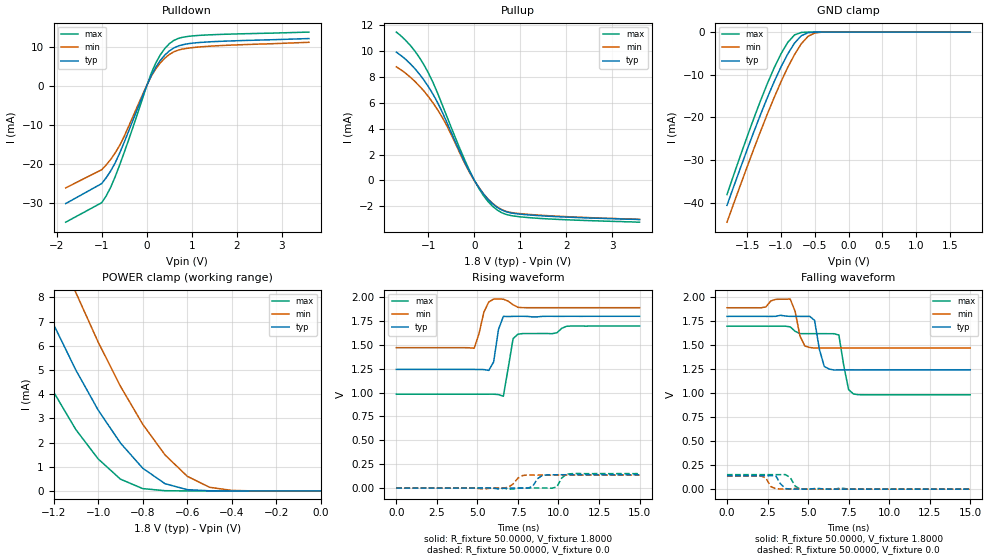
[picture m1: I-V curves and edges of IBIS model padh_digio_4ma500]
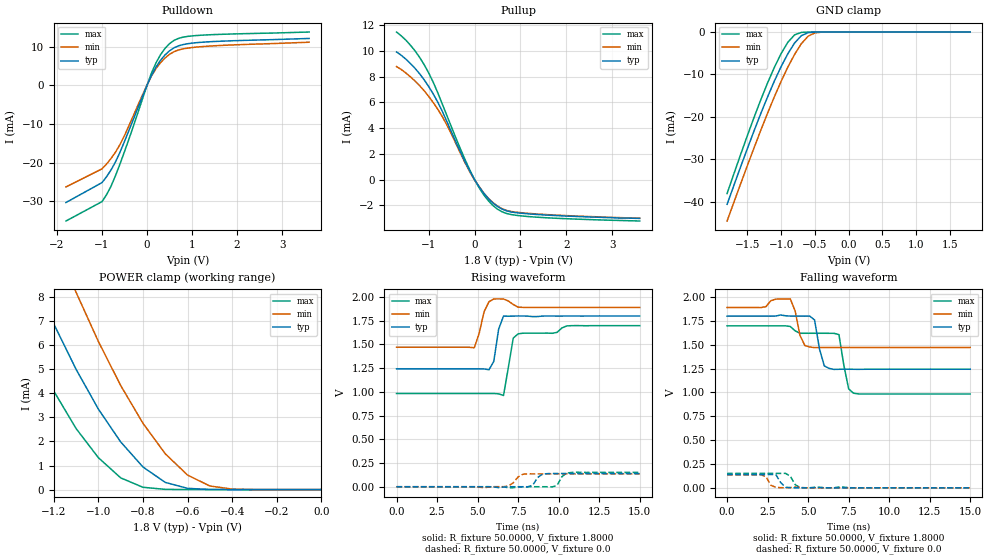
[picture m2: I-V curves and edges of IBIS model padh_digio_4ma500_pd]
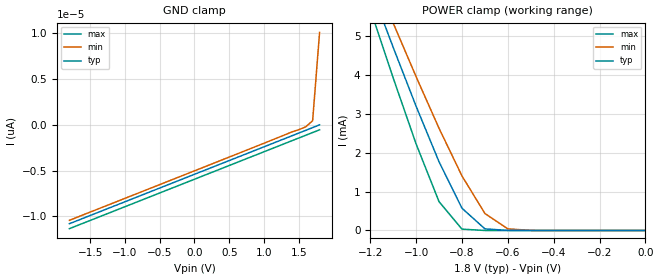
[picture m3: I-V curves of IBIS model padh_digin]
| IBIS file cs4272.ibs created by s2ibis3 verion 1.0
| North Carolina State University, ERL, 2005
[IBIS ver]   3.2
[Comment char]  |_char
[File name]   cs4272.ibs
[File Rev]   1.0B
[Date]   January 26, 2003
[Source]   HSpice Netlist
[Notes]   Rev. 1.0  1/26/2006  28-pin.  Original file.
|   Created by D. DeVries
[Copyright]   (C)opyright 2003 Cirrus Logic, Inc.  All Rights Reserved
[Component]   cs4272
[Manufacturer]  Cirrus Logic, Inc.
|   Component cs4272
[Package]
| variable   typ   min   max
R_pkg   12m   6.8m   16.1m
L_pkg   1.4n   0.713n   2.100n
C_pkg   0.27p   0.180p   0.368p
[Pin]  signal_name   model_name   R_pin   L_pin   C_pin
1   XTO   NC
2   XTI   NC
3   MCLK   padh_digio_mclk_pd
4   LRCK   padh_digio_4ma500
5   SCLK   padh_digio_4ma500
6   SDOUT   padh_digio_4ma500_pd
7   SDIN   padh_digin
8   DGND   GND
9   VD   POWER
10   VL   POWER
11   SCL_CCLK   padh_digin
12   SDA_CDIN   padh_digio_mclk
13   AD0_CSB   padh_digin
14   RSTB   padh_digin
15   VCOM   NC
16   AINA-   NC
17   AINA+   NC
18   AINB+   NC
19   AINB-   NC
20   VA   POWER
21   AGND   GND
22   FILT+   NC
23   AMUTECB   NC
24   AOUTA-   NC
25   AOUTA+   NC
26   AOUTB+   NC
27   AOUTB-   NC
28   BMUTECB   NC
| Models and submodels in the file (5): padh_digio_4ma500 (I/O), padh_digio_4ma500_pd (I/O), padh_digin (Input), padh_digio_mclk (I/O), padh_digio_mclk_pd (I/O)
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|   Model sclk
[Model]  padh_digio_4ma500
Model_type I/O
Polarity   Non-Inverting
Enable   Active-High
Vinl =   0.625V
Vinh =   0.975V
C_comp   5.0000pF   5.0000pF   5.0000pF
[Temperature Range]   25.0000   85.0000   -40.0000
[Voltage Range]   1.8000V   1.6200V   1.9800V
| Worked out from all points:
|   slope of the pulldown table from 0 to 0.27 V, typ, clamps not added: 45.5 ohm
|   slope of the pullup table from 0 to 0.27 V, typ, clamps not added: 199 ohm
|   GND clamp passes 1 mA (typ) near -0.71 V on its own axis
|   POWER clamp passes 1 mA (typ) near -0.81 V on its own axis
|   rising waveform, R_fixture 50.0000, V_fixture 1.8000: 20-80 % time 329ps typ, 374ps min, 423ps max; typ from 1.24 V to 1.8 V
|   rising waveform, R_fixture 50.0000, V_fixture 0.0: 20-80 % time 378ps typ, 473ps min, 360ps max; typ from 0 V to 0.139 V
|   falling waveform, R_fixture 50.0000, V_fixture 1.8000: 20-80 % time 401ps typ, 363ps min, 445ps max; typ from 1.8 V to 1.24 V
|   falling waveform, R_fixture 50.0000, V_fixture 0.0: 20-80 % time 366ps typ, 272ps min, 323ps max; typ from 0.139 V to 0 V
[Pulldown]
|Voltage   I(typ)   I(min)   I(max)
-1.8V     -30.27mA   -26.24mA   -35.05mA
-1V       -25.14mA   -21.58mA   -30.05mA
-900mV    -23.63mA   -20.35mA   -28.29mA
-800mV    -21.88mA   -18.91mA   -26.07mA
-600mV    -17.28mA   -15.3mA    -20.3mA
0V        -4.47pA    55.01uA    80fA
100mV     2.574mA    2.437mA    3.196mA
300mV     6.46mA     5.835mA    7.9mA
500mV     8.908mA    7.999mA    10.75mA
700mV     10.19mA    9.127mA    12.12mA
1.1V      11.01mA    9.864mA    12.85mA
3.6V      12.09mA    11.13mA    13.75mA
[Pullup]
|Voltage   I(typ)   I(min)   I(max)
-1.7V     9.93mA     8.79mA     11.48mA
-1.4V     9.04mA     8mA        10.47mA
-1.1V     7.773mA    6.922mA    8.954mA
-900mV    6.661mA    5.992mA    7.572mA
-700mV    5.289mA    4.882mA    5.856mA
-300mV    2.086mA    1.981mA    2.325mA
0V        110fA      -34.64uA   1.73pA
200mV     -1.061mA   -1.05mA    -1.188mA
500mV     -2.098mA   -2.065mA   -2.306mA
700mV     -2.441mA   -2.409mA   -2.646mA
1.2V      -2.681mA   -2.64mA    -2.89mA
3.6V      -3.04mA    -3.02mA    -3.24mA
[GND_clamp]
|Voltage   I(typ)   I(min)   I(max)
-1.8V     -40.64mA   -44.58mA   -38.09mA
-1.5V     -27.5mA    -31.52mA   -24.45mA
-1.3V     -19.19mA   -23.13mA   -15.94mA
-1.1V     -11.57mA   -15.28mA   -8.331mA
-1V       -8.145mA   -11.63mA   -5.085mA
-900mV    -5.12mA    -8.256mA   -2.402mA
-800mV    -2.575mA   -5.266mA   -663.9uA
-700mV    -853.9uA   -2.734mA   -79.03uA
-600mV    -146.2uA   -989.3uA   -4.169uA
-500mV    -12.66uA   -202.1uA   -123.3nA
-400mV    -717.4nA   -22.85uA   -2.457nA
1.8V      38.21pA    12.29nA    34.03pA
[POWER_clamp]
|Voltage   I(typ)   I(min)   I(max)
-1.8V     21.57mA    26.49mA    17.86mA
-1.4V     11.23mA    15.35mA    7.972mA
-1.3V     8.971mA    12.82mA    5.918mA
-1.2V     6.884mA    10.43mA    4.093mA
-1.1V     4.997mA    8.198mA    2.536mA
-1V       3.345mA    6.155mA    1.325mA
-900mV    1.981mA    4.328mA    487.2uA
-800mV    939.3uA    2.755mA    95.74uA
-700mV    299uA      1.489mA    9.484uA
-600mV    51.78uA    603.4uA    548.9nA
-400mV    325.5nA    21.08uA    346.2pA
0V        38.21pA    361.4pA    41.39pA
[Ramp]
| variable   typ   min   max
dV/dt_r  83.5800m/0.2801n   61.0800m/0.4049n   0.1165/0.2372n
dV/dt_f  0.3342/0.3283n   0.2298/0.4453n   0.4806/0.2633n
R_load = 50.0000
[Rising Waveform]
R_fixture= 50.0000
V_fixture= 1.8000
V_fixture_min= 1.9800
V_fixture_max= 1.6200
|time   V(typ)   V(min)   V(max)
0s        1.243V     1.471V     983.3mV
4.8ns     1.243V     1.465V     983.3mV
5.4ns     1.242V     1.845V     983.4mV
6ns       1.321V     1.98V      983.5mV
6.3ns     1.662V     1.98V      979.1mV
6.6ns     1.799V     1.98V      962mV
7.2ns     1.799V     1.921V     1.567V
7.5ns     1.8V       1.894V     1.613V
10.5ns    1.8V       1.89V      1.696V
15ns      1.8V       1.89V      1.698V
[Rising Waveform]
R_fixture= 50.0000
V_fixture= 0.0
|time   V(typ)   V(min)   V(max)
0s        0V         0V         0V
6.6ns     -3.12mV    20.98uV    -50.4uV
8.1ns     -958.2uV   136mV      -54.9uV
8.4ns     15.43mV    135.4mV    -17.87uV
9ns       131.7mV    135.4mV    7.61uV
9.6ns     138.8mV    135.6mV    -1.995mV
9.9ns     139.1mV    135.6mV    12.63mV
10.2ns    139.3mV    135.5mV    106mV
10.5ns    139.3mV    135.4mV    144.6mV
15ns      139.3mV    135.5mV    151.3mV
[Falling Waveform]
R_fixture= 50.0000
V_fixture= 1.8000
V_fixture_min= 1.9800
V_fixture_max= 1.6200
|time   V(typ)   V(min)   V(max)
0s        1.8V       1.89V      1.698V
3.9ns     1.8V       1.98V      1.691V
4.5ns     1.8V       1.596V     1.62V
5.1ns     1.8V       1.476V     1.62V
5.4ns     1.759V     1.47V      1.62V
6ns       1.278V     1.471V     1.62V
6.9ns     1.242V     1.471V     1.606V
7.5ns     1.243V     1.471V     1.037V
7.8ns     1.243V     1.471V     991.7mV
15ns      1.243V     1.471V     983.3mV
[Falling Waveform]
R_fixture= 50.0000
V_fixture= 0.0
|time   V(typ)   V(min)   V(max)
0s        139.3mV    135.5mV    151.2mV
2.1ns     139.3mV    136.7mV    151.2mV
2.4ns     139.2mV    116.2mV    151.2mV
2.7ns     139.8mV    26.37mV    151.2mV
3ns       140.4mV    5.168mV    151.2mV
3.3ns     55.83mV    1.512mV    151.1mV
3.9ns     1.888mV    1.869mV    121.8mV
4.2ns     470.2uV    7.829mV    32.89mV
4.5ns     168.8uV    3.003mV    2.446mV
15ns      -4.982uV   1.389uV    -6.351uV
|   Model sclk
[Model]  padh_digio_4ma500_pd
Model_type I/O
Polarity   Non-Inverting
Enable   Active-High
Vinl =   0.625V
Vinh =   0.975V
C_comp   5.0000pF   5.0000pF   5.0000pF
[Temperature Range]   25.0000   85.0000   -40.0000
[Voltage Range]   1.8000V   1.6200V   1.9800V
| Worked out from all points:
|   slope of the pulldown table from 0 to 0.27 V, typ, clamps not added: 45.5 ohm
|   slope of the pullup table from 0 to 0.27 V, typ, clamps not added: 200 ohm
|   GND clamp passes 1 mA (typ) near -0.71 V on its own axis
|   POWER clamp passes 1 mA (typ) near -0.81 V on its own axis
|   rising waveform, R_fixture 50.0000, V_fixture 1.8000: 20-80 % time 329ps typ, 374ps min, 423ps max; typ from 1.24 V to 1.8 V
|   rising waveform, R_fixture 50.0000, V_fixture 0.0: 20-80 % time 382ps typ, 475ps min, 363ps max; typ from 0 V to 0.139 V
|   falling waveform, R_fixture 50.0000, V_fixture 1.8000: 20-80 % time 401ps typ, 363ps min, 445ps max; typ from 1.8 V to 1.24 V
|   falling waveform, R_fixture 50.0000, V_fixture 0.0: 20-80 % time 367ps typ, 274ps min, 327ps max; typ from 0.139 V to 0 V
[Pulldown]
|Voltage   I(typ)   I(min)   I(max)
-1.8V     -30.27mA   -26.24mA   -35.05mA
-1V       -25.13mA   -21.58mA   -30.04mA
-900mV    -23.63mA   -20.35mA   -28.29mA
-800mV    -21.87mA   -18.91mA   -26.07mA
-600mV    -17.28mA   -15.3mA    -20.29mA
0V        -4.47pA    55.01uA    80fA
100mV     2.574mA    2.437mA    3.196mA
300mV     6.46mA     5.836mA    7.9mA
500mV     8.908mA    7.999mA    10.75mA
700mV     10.19mA    9.127mA    12.12mA
1.1V      11.01mA    9.864mA    12.85mA
3.6V      12.09mA    11.12mA    13.75mA
[Pullup]
|Voltage   I(typ)   I(min)   I(max)
-1.7V     9.93mA     8.79mA     11.48mA
-1.4V     9.04mA     8mA        10.47mA
-1.1V     7.772mA    6.921mA    8.953mA
-900mV    6.661mA    5.992mA    7.572mA
-700mV    5.288mA    4.882mA    5.856mA
-300mV    2.086mA    1.981mA    2.325mA
0V        0A         -34.64uA   0A
200mV     -1.061mA   -1.051mA   -1.189mA
500mV     -2.098mA   -2.065mA   -2.306mA
700mV     -2.441mA   -2.409mA   -2.646mA
1.2V      -2.681mA   -2.641mA   -2.89mA
3.6V      -3.03mA    -3.01mA    -3.23mA
[GND_clamp]
|Voltage   I(typ)   I(min)   I(max)
-1.8V     -40.65mA   -44.58mA   -38.1mA
-1.5V     -27.51mA   -31.52mA   -24.45mA
-1.3V     -19.19mA   -23.13mA   -15.94mA
-1.1V     -11.57mA   -15.28mA   -8.334mA
-1V       -8.147mA   -11.63mA   -5.087mA
-900mV    -5.122mA   -8.258mA   -2.404mA
-800mV    -2.577mA   -5.267mA   -665.9uA
-700mV    -855.3uA   -2.736mA   -80.74uA
-600mV    -147.4uA   -990.4uA   -5.602uA
-500mV    -13.65uA   -203uA     -1.287uA
-400mV    -1.484uA   -23.55uA   -906.2nA
1.8V      662.4nA    593.8nA    803nA
[POWER_clamp]
|Voltage   I(typ)   I(min)   I(max)
-1.8V     21.57mA    26.49mA    17.86mA
-1.4V     11.23mA    15.35mA    7.973mA
-1.3V     8.972mA    12.82mA    5.919mA
-1.2V     6.884mA    10.43mA    4.094mA
-1.1V     4.998mA    8.199mA    2.537mA
-1V       3.345mA    6.155mA    1.326mA
-900mV    1.982mA    4.328mA    488uA
-800mV    939.9uA    2.756mA    96.54uA
-700mV    299.6uA    1.49mA     10.29uA
-600mV    52.45uA    603.9uA    1.354uA
-400mV    988.9nA    21.66uA    804.8nA
0V        662.4nA    581.4nA    803.5nA
[Ramp]
| variable   typ   min   max
dV/dt_r  83.5800m/0.2811n   61.0800m/0.4067n   0.1165/0.2408n
dV/dt_f  0.3342/0.3283n   0.2298/0.4456n   0.4806/0.2633n
R_load = 50.0000
[Rising Waveform]
R_fixture= 50.0000
V_fixture= 1.8000
V_fixture_min= 1.9800
V_fixture_max= 1.6200
|time   V(typ)   V(min)   V(max)
0s        1.243V     1.471V     983.3mV
4.8ns     1.243V     1.465V     983.3mV
5.4ns     1.242V     1.844V     983.3mV
6ns       1.321V     1.98V      983.4mV
6.3ns     1.662V     1.98V      979.1mV
6.6ns     1.799V     1.979V     961.9mV
7.2ns     1.799V     1.921V     1.567V
7.5ns     1.8V       1.893V     1.612V
10.5ns    1.8V       1.89V      1.696V
15ns      1.8V       1.89V      1.698V
[Rising Waveform]
R_fixture= 50.0000
V_fixture= 0.0
|time   V(typ)   V(min)   V(max)
0s        0V         0V         0V
6.6ns     -3.209mV   18.89uV    -48.55uV
8.1ns     -939.6uV   135.9mV    -56.57uV
8.4ns     15.3mV     135.4mV    -19.32uV
9ns       131.4mV    135.4mV    7.337uV
9.6ns     138.8mV    135.6mV    -1.966mV
9.9ns     139.1mV    135.6mV    12.47mV
10.2ns    139.3mV    135.5mV    105.4mV
10.5ns    139.3mV    135.4mV    144.4mV
15ns      139.3mV    135.5mV    151.3mV
[Falling Waveform]
R_fixture= 50.0000
V_fixture= 1.8000
V_fixture_min= 1.9800
V_fixture_max= 1.6200
|time   V(typ)   V(min)   V(max)
0s        1.8V       1.89V      1.698V
3.9ns     1.8V       1.98V      1.691V
4.5ns     1.8V       1.596V     1.62V
5.1ns     1.8V       1.476V     1.62V
5.4ns     1.759V     1.47V      1.62V
6ns       1.278V     1.471V     1.62V
6.9ns     1.242V     1.471V     1.606V
7.5ns     1.243V     1.471V     1.037V
7.8ns     1.242V     1.471V     991.7mV
15ns      1.243V     1.471V     983.3mV
[Falling Waveform]
R_fixture= 50.0000
V_fixture= 0.0
|time   V(typ)   V(min)   V(max)
0s        139.3mV    135.5mV    151.2mV
2.1ns     139.3mV    136.7mV    151.2mV
2.4ns     139.2mV    116.5mV    151.2mV
2.7ns     139.7mV    27.16mV    151.2mV
3ns       140.5mV    5.372mV    151.2mV
3.3ns     56.63mV    1.575mV    151.1mV
3.9ns     1.953mV    1.849mV    122.1mV
4.2ns     490.1uV    7.789mV    33.45mV
4.5ns     174.6uV    3.031mV    2.607mV
15ns      -4.339uV   1.407uV    -11.58uV
|   Model padh_digin
[Model]  padh_digin
Model_type Input
Vinl =   0.6250V
Vinh =   0.9750V
C_comp   5.0000pF   5.0000pF   5.0000pF
[Temperature Range]   25.0000   85.0000   -40.0000
[Voltage Range]   1.8000V   1.6200V   1.9800V
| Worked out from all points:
|   POWER clamp passes 1 mA (typ) near -0.84 V on its own axis
[GND_clamp]
|Voltage   I(typ)   I(min)   I(max)
-1.8V     -10.8pA    -10.43pA   -11.34pA
1.6V      -600.1fA   -217.6fA   -1.14pA
1.7V      -300.1fA   450.2fA    -840fA
1.8V      0A         10.1pA     -540fA
[POWER_clamp]
|Voltage   I(typ)   I(min)   I(max)
-1.8V     15.99mA    15.48mA    16.76mA
-1.2V     6.274mA    6.747mA    5.694mA
-1.1V     4.711mA    5.337mA    3.925mA
-1V       3.195mA    3.956mA    2.226mA
-900mV    1.767mA    2.629mA    741.3uA
-800mV    572.3uA    1.403mA    34.11uA
-700mV    41.8uA     437uA      266.3nA
-600mV    967.8nA    41.61uA    1.853nA
-500mV    19.92nA    1.821uA    14.35pA
0V        0A         0A         0A
